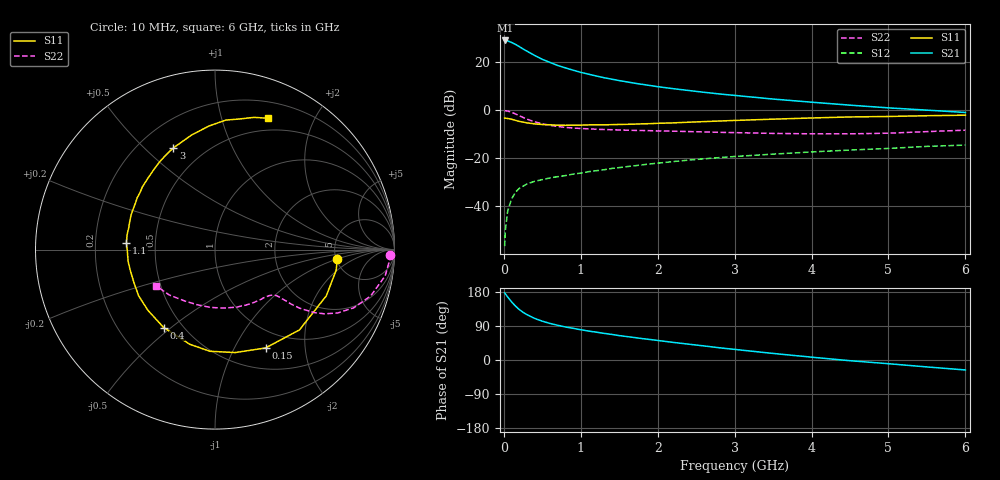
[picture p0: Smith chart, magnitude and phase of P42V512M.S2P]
! SIEMENS Small Signal Semiconductors
! BFP182
! Si NPN RF Bipolar Junction Transistor in SOT143
! VCE = 2.5 V  IC = 12 mA
! Common Emitter S-Parameters:  March  1996
# GHz  S  MA  R  50
!  f  S11  S21  S12  S22
! GHz  MAG  ANG  MAG  ANG  MAG  ANG  MAG  ANG
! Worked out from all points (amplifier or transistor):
!   36 points, 10 MHz to 6 GHz, reference 50 ohm
!   highest |S21| = 29.0 dB at 20 MHz (marker M1)
!   |S21| within 3 dB of that: start of sweep to 223.2 MHz
!   unconditionally stable (mu >= 1): 1.004 GHz to 5.369 GHz
!   at 250 MHz: K = 0.38, MSG = 28.5 dB, |S12| = -31.6 dB
!   at 1.4 GHz: K = 1.10, MAG = 16.6 dB, |S12| = -24.2 dB
!   at 6 GHz: K = 0.93, MSG = 6.8 dB, |S12| = -14.5 dB
!   S11 on the Smith chart (normalised r, x): 10 MHz: 5.10, -1.02; 150 MHz: 0.76, -1.34; 400 MHz: 0.40, -0.47; 1.1 GHz: 0.34, +0.03; 3 GHz: 0.34, +0.62; 6 GHz: 0.37, +1.41
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0.01  0.683 -4.5  27.84 177.3  0.0015 79.7  0.9781 -1.6
0.02  0.6849 -9.6  28.08 174.7  0.0032 79.7  0.9745 -3.5
0.05  0.6715 -22.6  27.46 166.2  0.0081 82.3  0.9593 -8.8
0.1  0.6492 -43.6  25.54 153.6  0.0142 70.0  0.905 -16.6
0.15  0.6161 -62.8  23.34 142.5  0.0197 62.6  0.8377 -22.8
0.2  0.5846 -78.9  20.98 133.3  0.0238 58.0  0.7696 -27.3
0.25  0.5672 -92.8  18.68 125.8  0.0264 53.3  0.7074 -30.4
0.3  0.5461 -104.8  16.84 119.8  0.0294 50.6  0.6528 -32.5
0.4  0.5199 -123.4  13.73 109.8  0.0333 48.2  0.5735 -34.7
0.5  0.5041 -137.8  11.4 102.4  0.0362 45.6  0.5211 -35.6
0.6  0.4973 -148.9  9.819 96.5  0.0392 45.9  0.4848 -35.9
0.7  0.4875 -158.0  8.484 91.6  0.0417 45.6  0.459 -36.3
0.9  0.4885 -172.2  6.782 83.6  0.0471 46.3  0.4268 -36.9
1.1  0.4952 175.5  5.604 76.4  0.0528 47.0  0.4091 -38.3
1.5  0.5058 157.6  4.123 64.4  0.0642 47.6  0.3887 -42.4
1.8  0.5212 146.2  3.44 56.5  0.0733 46.7  0.3786 -46.6
2.2  0.5452 133.5  2.801 46.5  0.0856 45.3  0.3669 -53.1
3  0.6124 112.2  2.028 28.0  0.1093 39.9  0.3424 -69.5
3.5  0.6514 101.6  1.704 17.3  0.1224 36.0  0.3294 -81.5
4.5  0.7241 85.2  1.272 -1.9  0.1487 28.3  0.3229 -108.4
5.5  0.768 73.6  1.003 -18.3  0.1771 20.6  0.3591 -135.3
6  0.7883 68.2  0.897 -26.3  0.1885 15.8  0.3846 -148.0
